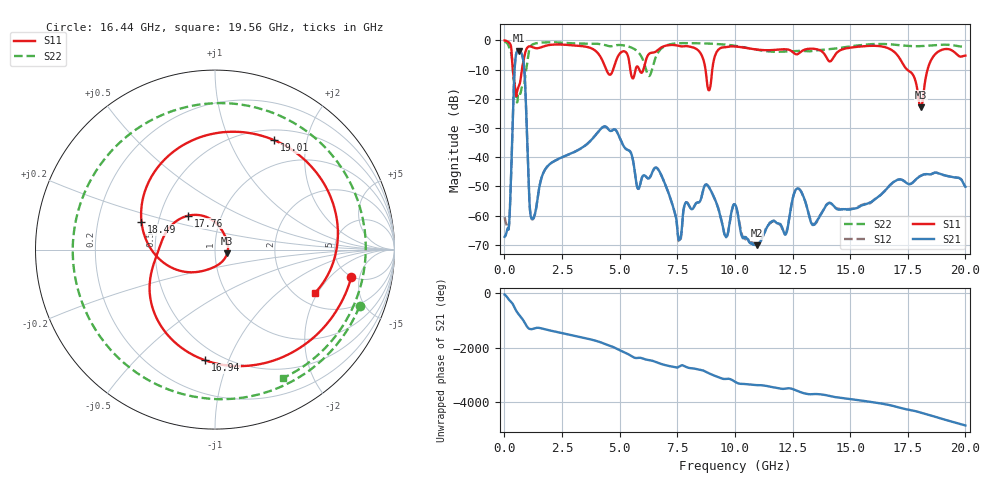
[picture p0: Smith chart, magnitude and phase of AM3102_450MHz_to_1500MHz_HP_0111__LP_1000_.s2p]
!Agilent Technologies,E8364B,MY43040894,A.07.50.67
!Agilent E8364B: A.07.50.67
!Date: Thursday, January 11, 2018 05:53:03
!Correction: S11(Full 2 Port(1,2))
!S21(Full 2 Port(1,2))
!S12(Full 2 Port(1,2))
!S22(Full 2 Port(1,2))
!S2P File: Measurements: S11, S21, S12, S22:
# Hz S  dB  R 50
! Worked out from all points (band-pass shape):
!   1601 points, 10 MHz to 20 GHz, reference 50 ohm
!   highest |S21| = -3.53 dB at 622.2 MHz (marker M1); lowest = -70.1 dB at 10.94 GHz (marker M2)
!   |S21| within 3 dB of the highest: 476.3 MHz to 812.8 MHz (336.6 MHz wide, 52.2 % of centre)
!   lowest |S11| = -22.9 dB at 18.06 GHz (marker M3), VSWR 1.15, Z = 57.3 - j2.32 ohm
!   |S11| at or under -10 dB: 368.6 MHz to 758.1 MHz (389.4 MHz wide, 69.1 % of centre); 4.419 GHz to 4.719 GHz (299.9 MHz wide, 6.56 % of centre); 17.47 GHz to 18.36 GHz (892.4 MHz wide, 4.98 % of centre)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
!   |S22| runs from -21.2 to -0.4 dB; largest |S21 - S12| = 0.0013
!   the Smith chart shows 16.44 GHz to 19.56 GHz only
!   S11 on the Smith chart (normalised r, x): 16.44 GHz: 4.91, -3.77; 16.94 GHz: 0.41, -0.83; 17.76 GHz: 0.69, +0.28; 18.49 GHz: 0.40, +0.15; 19.01 GHz: 0.63, +1.49; 19.56 GHz: 2.50, -1.89
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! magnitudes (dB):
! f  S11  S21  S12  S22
! 10 MHz  -0.1  -67.2  -60.5  -0.4
! 197.4 MHz  -0.7  -63.7  -63.6  -2.3
! 447.3 MHz  -15.2  -9.4  -9.4  -15.5
! 622.2 MHz  -15.8  -3.5  -3.5  -17.8
! 847.1 MHz  -6.3  -8.5  -8.5  -15.4
! 1.209 GHz  -2.3  -61.1  -61.3  -1.5
! 3.346 GHz  -2.0  -36.9  -36.9  -1.1
! 6.682 GHz  -3.2  -44.3  -44.3  -4.0
! 7.594 GHz  -2.0  -68.4  -69.1  -1.0
! 8.881 GHz  -17.1  -50.3  -50.3  -1.1
! 10.01 GHz  -2.1  -56.2  -56.2  -1.9
! 10.94 GHz  -3.2  -70.1  -70.4  -3.2
! 13.34 GHz  -2.9  -62.9  -62.3  -3.7
! 16.44 GHz  -2.2  -52.0  -52.1  -1.3
! 16.68 GHz  -2.8  -50.0  -50.0  -1.4
! 16.94 GHz  -4.2  -48.2  -48.2  -1.5
! 17.76 GHz  -12.4  -48.3  -48.3  -2.0
! 18.06 GHz  -22.9  -46.4  -46.3  -2.0
! 18.49 GHz  -7.2  -45.9  -45.9  -1.8
! 19.01 GHz  -3.2  -46.0  -46.0  -1.5
! 19.56 GHz  -4.3  -47.0  -46.9  -1.8
! 20 GHz  -5.2  -50.1  -50.2  -2.4
